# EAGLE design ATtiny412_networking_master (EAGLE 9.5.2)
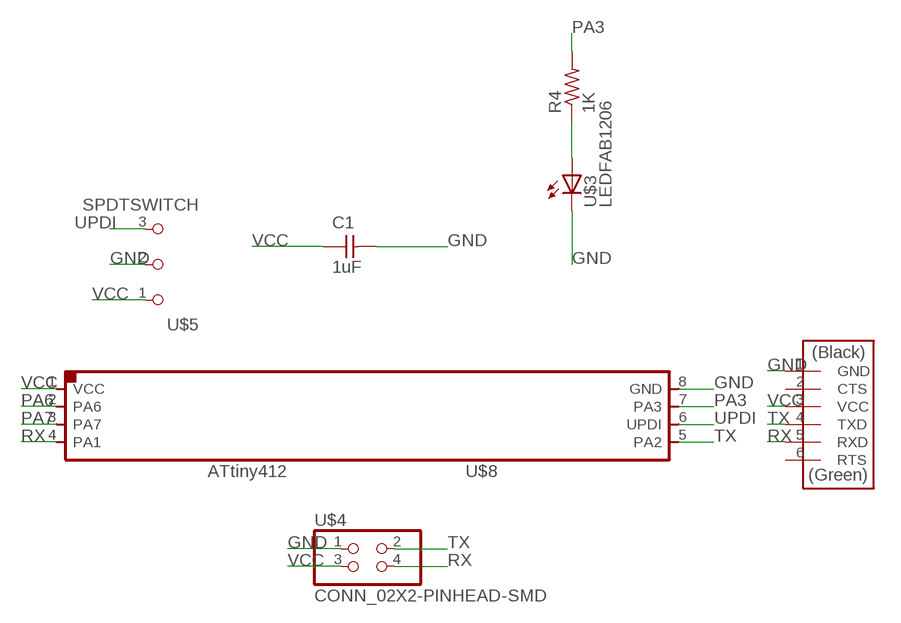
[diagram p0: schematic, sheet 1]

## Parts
C1  1uF  CAP_UNPOLARIZEDFAB  [C1206FAB]
R4  1K  R1206FAB  [R1206FAB]
U$2  CONN_06_FTDI-SMD-HEADER  [1X06SMD]
U$3  LEDFAB1206  [LED1206FAB]
U$4  CONN_02X2-PINHEAD-SMD  [2X02SMD]
U$5  SPDTSWITCH  [SPDTSWITCH]
U$8  UC_ATTINY45SI  [SOIC8]

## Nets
GND: C1.2 U$2.1(GND) U$3.2(C) U$4.1 U$5.2 U$8.8(GND)
N$1: R4.1 U$3.1(A)
PA3: R4.2 U$8.7(PA3)
PA6: U$8.2(PA6)
PA7: U$8.3(PA7)
RX: U$2.5(RXD) U$4.4 U$8.4(PA1)
TX: U$2.4(TXD) U$4.2 U$8.5(PA2)
UPDI: U$5.3 U$8.6(UPDI)
VCC [New Class]: C1.1 U$2.3(VCC) U$4.3 U$5.1 U$8.1(VCC)
Unconnected: U$2.2(CTS) U$2.6(RTS)

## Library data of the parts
C1 = fab:CAP_UNPOLARIZED
R4 = fab:R: Resistor (US Symbol)
U$2 = fab:CONN_06_FTDI-SMD-HEADER
U$3 = fab:LED: LED
U$4 = fab:CONN_02X2-PINHEAD-SMD
U$5 = fab:SPDTSWITCH
U$8 = fab:UC_ATTINY45

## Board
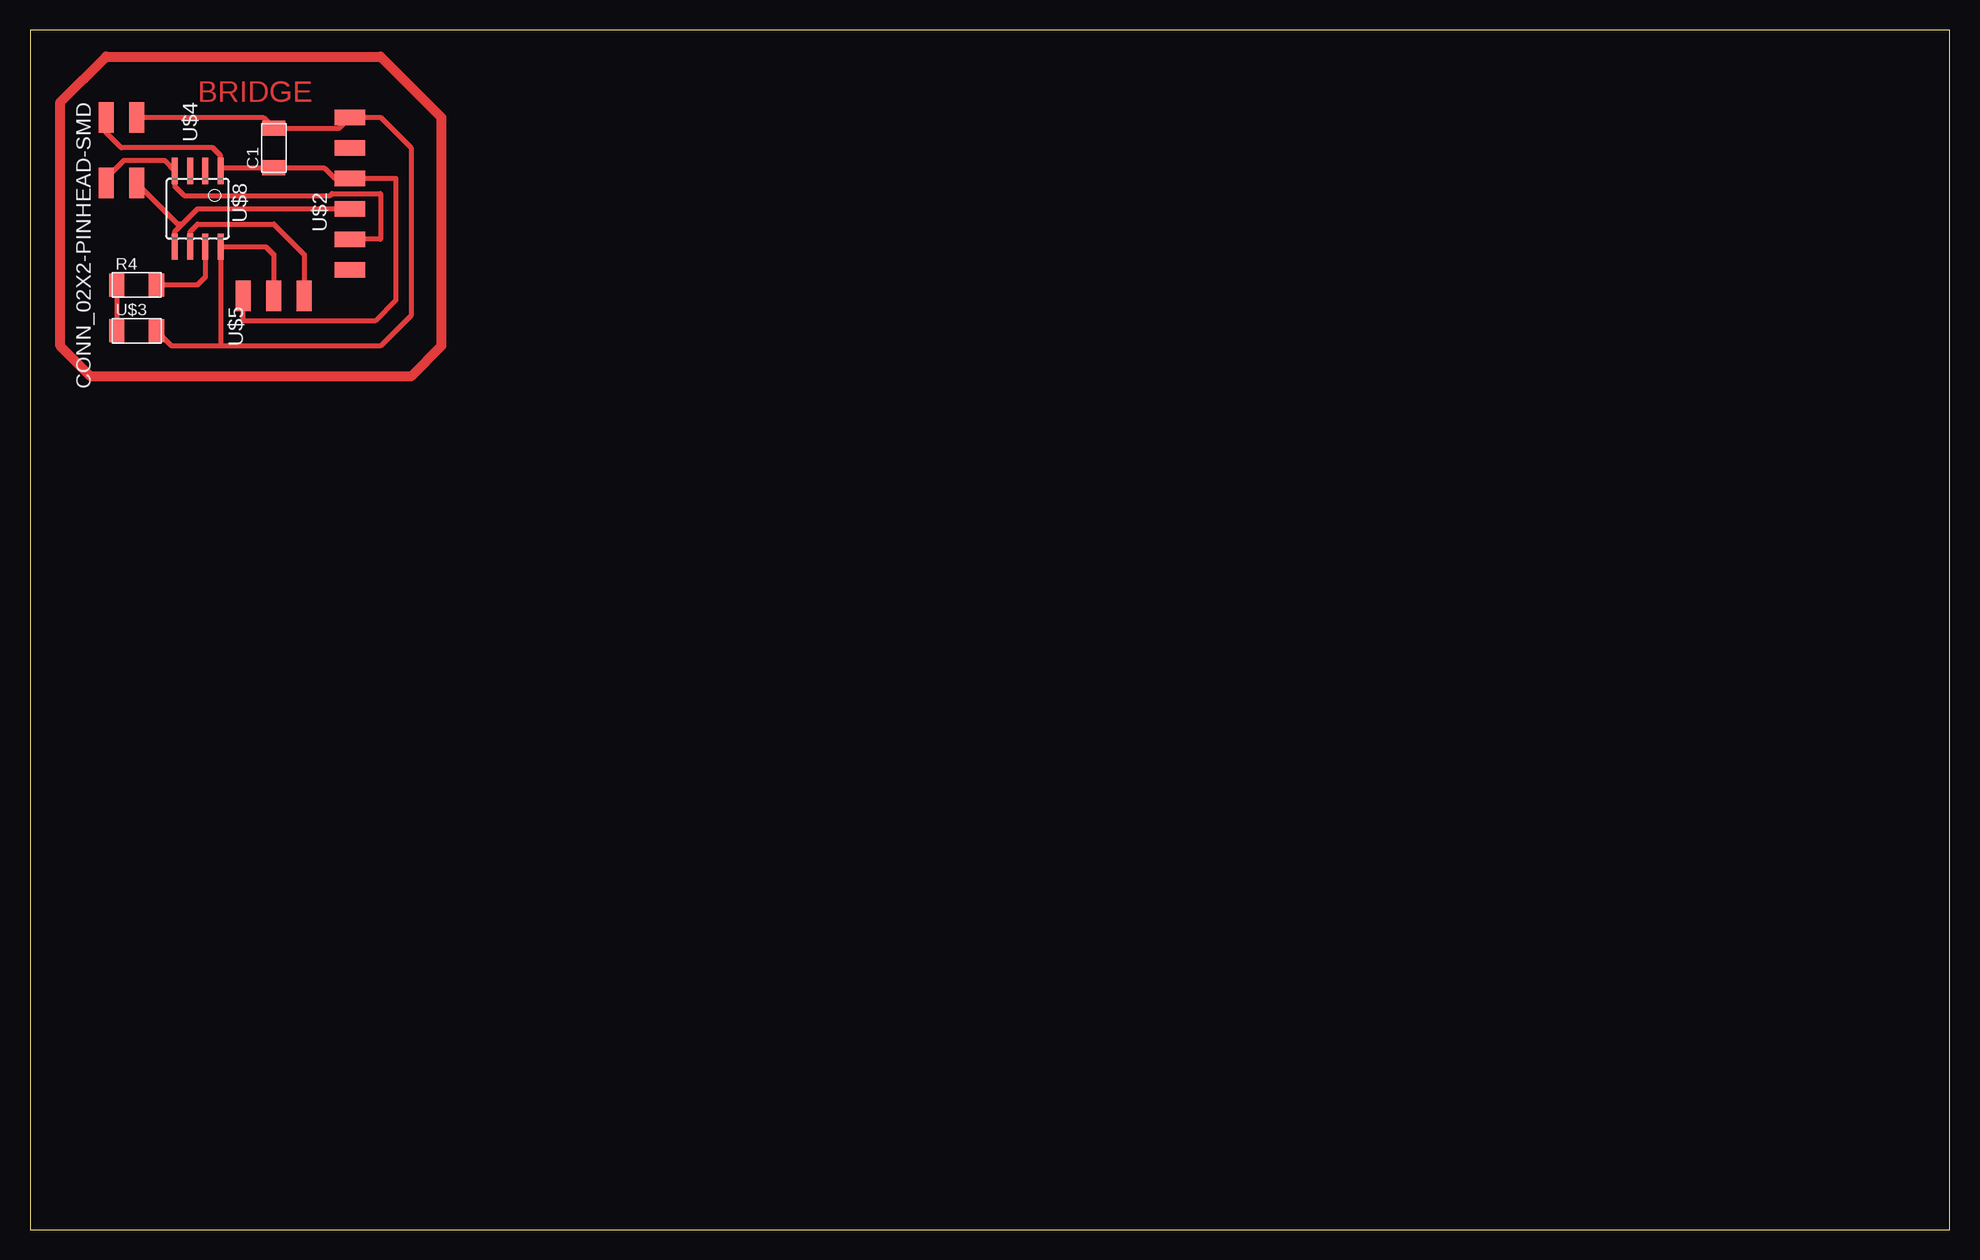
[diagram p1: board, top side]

Size 160 x 100 mm. Coordinates in mm from the lower left corner, seen from the top.
Outline: 0,0 160,0 160,100 0,100 0,0
Copper layers (1*16): Top 0.035mm / dielectric 1.5mm / Bottom 0.035mm
Design rules "default *": minimum track width 16mil, minimum drill 0.35mm, track to track 16mil, track to pad 16mil, pad to pad 16mil, via to via 16mil, smd to smd 6mil, copper to edge 40mil, drill to drill 6mil, minimum pad ring 10mil, minimum via ring 8mil, stop-mask expansion 4mil, vias tented up to drill 0mil, thermal gap 10mil

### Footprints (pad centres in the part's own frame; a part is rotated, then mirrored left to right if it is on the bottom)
C1206FAB = smd 1.27 x 1.905: 1 -1.651,0; 2 1.651,0
R1206FAB = smd 1.27 x 1.905: 1 -1.651,0; 2 1.651,0
1X06SMD = smd 2.54 x 1.27: 1 0,6.35; 2 0,3.81; 3 0,1.27; 4 0,-1.27; 5 0,-3.81; 6 0,-6.35
LED1206FAB = smd 1.27 x 1.905: 1 -1.651,0; 2 1.651,0
2X02SMD = smd 2.54 x 1.27: 1 -2.54,1.27; 2 2.92,1.27; 3 -2.54,-1.27; 4 2.92,-1.27
SPDTSWITCH = smd 2.54 x 1.27: 1 0.38,2.54; 2 0.38,0; 3 0.38,-2.54
SOIC8 = smd 0.5 x 2.2: 1 -1.905,-3.154; 2 -0.645,-3.154; 3 0.625,-3.154; 4 1.895,-3.154; 5 1.905,3.154; 6 0.635,3.154; 7 -0.635,3.154; 8 -1.905,3.154

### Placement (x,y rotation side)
C1  20.32,90.17 90 top
R4  8.89,78.74 0 top
U$2  26.67,86.36 0 top
U$3  8.89,74.93 0 top
U$4  7.62,90.17 270 top
U$5  20.32,77.47 90 top
U$8  13.97,85.09 180 top

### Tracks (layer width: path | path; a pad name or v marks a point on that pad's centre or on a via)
GND
  Top 0.406: C1.2 25.78,91.82 U$2.1 29.21,92.71 31.75,90.17 31.75,76.2 29.21,73.66 15.88,73.66 | 20.6,92.1 C1.2 | 15.88,73.66 11.81,73.66 U$3.2 | U$4.1 19.43,92.71 C1.2 | U$5.2 20.32,81.28 19.66,81.94 U$8.8 15.88,73.66
N$1
  Top 0.406: R4.1 U$3.1
N$2
  Top 0.813: 34.29,73.66 31.75,71.12 5.08,71.12 2.54,73.66 2.54,93.98 6.35,97.79 29.21,97.79 34.29,92.71 34.29,73.66
PA3
  Top 0.406: U$8.7 14.61,79.4 13.95,78.74 R4.2
RX
  Top 0.406: U$2.5 29.21,82.55 29.21,86.36 25.17,86.36 25.02,86.21 12.85,86.21 12.07,86.98 U$8.4 11.19,89.13 7.85,89.13 6.35,87.63 U$4.4
TX
  Top 0.406: U$8.5 12.06,83.19 12.7,83.82 | 12.7,83.82 13.97,85.09 U$2.4 25.4,85.09 | 12.7,83.82 12.32,83.82 U$4.2
UPDI
  Top 0.406: U$8.6 13.34,83.19 13.97,83.82 20.32,83.82 22.86,81.28 U$5.3
VCC
  Top 0.406: C1.1 16.15,88.52 U$8.1 15.88,89.53 15.24,90.17 7.62,90.17 6.35,91.44 U$4.3 | C1.1 20.7,88.9 | C1.1 24.51,88.52 25.4,87.63 U$2.3 30.48,87.63 30.48,77.47 28.75,75.74 17.78,75.74 U$5.1

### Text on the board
Top: BRIDGE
